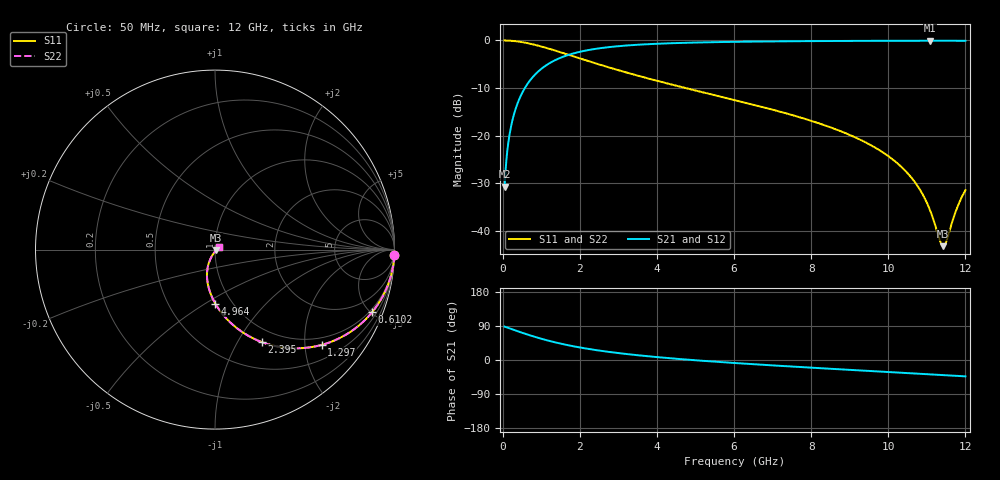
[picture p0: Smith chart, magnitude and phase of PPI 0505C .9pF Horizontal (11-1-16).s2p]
# MHz S MA R 50
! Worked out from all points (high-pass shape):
!   1601 points, 50 MHz to 12 GHz, reference 50 ohm
!   highest |S21| = -0.07 dB at 11.09 GHz (marker M1); lowest = -30.8 dB at 50 MHz (marker M2)
!   |S21| within 3 dB of the highest: 1.695 GHz to end of sweep
!   lowest |S11| = -43.2 dB at 11.42 GHz (marker M3), VSWR 1.01, Z = 50.5 - j0.456 ohm
!   |S11| at or under -10 dB: 4.741 GHz to end of sweep
!   |S22| runs from -43.2 to 0.0 dB; largest |S21 - S12| = 0
!   S11 on the Smith chart (normalised r, x): 50 MHz: 1, -62; 610.2 MHz: 0.82, -5.09; 1.297 GHz: 0.82, -2.38; 2.395 GHz: 0.82, -1.27; 4.964 GHz: 0.84, -0.55; 12 GHz: 1.05, +0.03
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50  0.9996 -1.8  0.02896 88.2  0.02896 88.2  0.9996 -1.8
154.5625  0.996 -5.7  0.08921 84.3  0.08921 84.3  0.996 -5.7
251.6562  0.9895 -9.2  0.1443 80.8  0.1443 80.8  0.9895 -9.2
408.5  0.973 -14.8  0.2304 75.2  0.2304 75.2  0.973 -14.8
610.1562  0.9425 -21.7  0.3336 68.3  0.3336 68.3  0.9425 -21.7
908.9062  0.8839 -31.1  0.4666 58.8  0.4666 58.8  0.8839 -31.1
1297.281  0.7972 -41.7  0.6021 48.1  0.6021 48.1  0.7972 -41.7
2044.156  0.6393 -57.5  0.7666 32.3  0.7666 32.3  0.6393 -57.5
2395.188  0.5767 -63.2  0.8144 26.5  0.8144 26.5  0.5767 -63.2
4038.312  0.3733 -82.2  0.9241 7.3  0.9241 7.3  0.3733 -82.2
4964.438  0.3004 -89.7  0.9497 -0.4  0.9497 -0.4  0.3004 -89.7
6025  0.236 -97.0  0.9671 -8.0  0.9671 -8.0  0.236 -97.0
8019.156  0.1423 -108.3  0.9842 -20.4  0.9842 -20.4  0.1423 -108.3
9169.344  0.09475 -113.6  0.9893 -27.0  0.9893 -27.0  0.09475 -113.6
10013.31  0.06033 -116.0  0.9915 -31.8  0.9915 -31.8  0.06033 -116.0
10655.62  0.03387 -114.5  0.9924 -35.4  0.9924 -35.4  0.03387 -114.5
11088.81  0.01622 -103.6  0.9925 -37.9  0.9925 -37.9  0.01622 -103.6
11342.75  0.007793 -68.0  0.9925 -39.4  0.9925 -39.4  0.007793 -68.0
11424.91  0.006889 -40.9  0.9924 -39.8  0.9924 -39.8  0.006889 -40.9
11514.53  0.007927 -11.5  0.9924 -40.4  0.9924 -40.4  0.007927 -11.5
11813.28  0.01861 25.4  0.992 -42.1  0.992 -42.1  0.01861 25.4
12000  0.02668 31.1  0.9917 -43.2  0.9917 -43.2  0.02668 31.1
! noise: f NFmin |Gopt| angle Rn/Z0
50  0.001231  0.9722  1.465  0.01005
1372  0.005838  0.7712  7.496  0.005181
2701  0.009172  0.7181  11.81  0.00637
4031  0.01212  0.6877  16.24  0.007398
5360  0.0149  0.6679  20.66  0.00835
6682  0.01758  0.655  25.01  0.009276
8012  0.02028  0.647  29.31  0.01023
9341  0.02301  0.6429  33.5  0.01122
1.067e+04  0.02583  0.6422  37.58  0.0123
1.2e+04  0.02879  0.6443  41.54  0.01348
